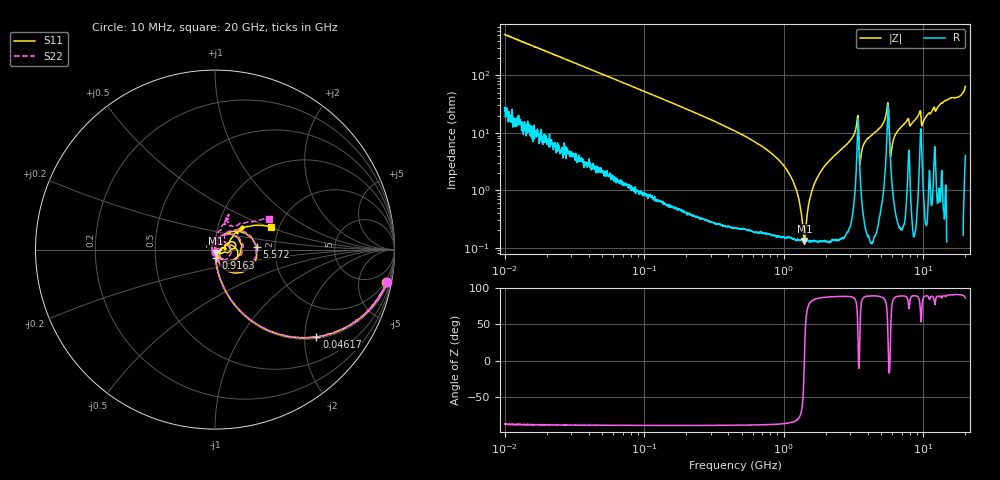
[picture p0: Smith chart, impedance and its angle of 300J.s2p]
!Keysight Technologies,P5008B,MY61100088,A.16.20.02
!Date: Tuesday, November 07, 2023 15:58:33
!Correction: S11(C  2-Port  )
!S21(C  2-Port  )
!S12(C  2-Port  )
!S22(C  2-Port  )
!S2P File: Measurements: S11, S21, S12, S22:Log Frequency Sweep
# Hz S  dB  R 50
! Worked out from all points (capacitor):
!   1601 points, 10 MHz to 20 GHz, reference 50 ohm
!   read as one part in series: C = 30.7 pF near 10.39 MHz
!   lowest |Z| = 130 mohm at 1.405 GHz (marker M1)
!   series resonance near 1.403 GHz, so ESL is about 420 pH
!   S11 on the Smith chart (normalised r, x): 10 MHz: 2, -10; 46.17 MHz: 1.04, -2.28; 916.3 MHz: 1.00, -0.09; 5.572 GHz: 1.60, +0.05; 20 GHz: 1.81, +0.52
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1e7  -0.24 -10.8  -14.53 76.2  -14.53 76.2  -0.24 -10.8
3.555162e7  -1.73 -33.8  -5.11 54.9  -5.11 54.9  -1.73 -33.8
4.616707e7  -2.54 -40.8  -3.71 48.2  -3.71 48.1  -2.55 -40.8
1.263918e8  -8.30 -66.7  -0.75 22.4  -0.75 22.4  -8.30 -66.7
4.472136e8  -18.93 -83.1  -0.07 5.8  -0.08 5.8  -18.92 -83.0
9.163254e8  -26.72 -86.3  -0.02 1.2  -0.02 1.2  -26.71 -87.3
1.405182e9  -34.61 -81.1  -0.01 -1.1  -0.01 -1.1  -34.60 -92.6
1.589917e9  -38.59 -75.5  -0.01 -1.8  -0.01 -1.8  -38.69 -94.4
1.807504e9  -44.40 -55.7  -0.01 -2.5  -0.01 -2.5  -45.47 -100.3
2.006635e9  -49.29 10.9  -0.01 -3.2  -0.01 -3.2  -65.21 138.1
2.30303e9  -41.98 71.1  -0.01 -4.2  -0.01 -4.2  -43.21 75.9
3.33599e9  -20.05 58.0  -0.38 -10.8  -0.39 -10.8  -19.80 53.7
3.721149e9  -41.85 99.7  -0.03 -6.6  -0.03 -6.6  -38.24 27.0
5.572426e9  -12.67 3.4  -2.13 -15.2  -2.13 -15.2  -12.77 6.2
5.652411e9  -14.01 -39.3  -1.57 -4.7  -1.57 -4.7  -14.27 -37.6
6.395515e9  -32.55 -40.4  -0.01 -12.0  -0.01 -12.0  -38.26 -147.9
7.552409e9  -25.68 18.0  -0.03 -16.5  -0.03 -16.5  -28.26 111.4
8.226633e9  -30.15 -26.3  -0.01 -16.9  -0.01 -16.9  -35.50 175.0
9.441767e9  -20.24 14.2  -0.42 -23.5  -0.42 -23.5  -23.34 42.4
1.038284e10  -30.06 -18.0  0.01 -21.8  0.01 -21.8  -34.66 152.6
1.367661e10  -16.18 38.0  -0.16 -29.9  -0.16 -29.9  -16.47 68.9
2e10  -9.43 22.1  -0.97 -57.5  -0.98 -57.4  -9.21 29.9
